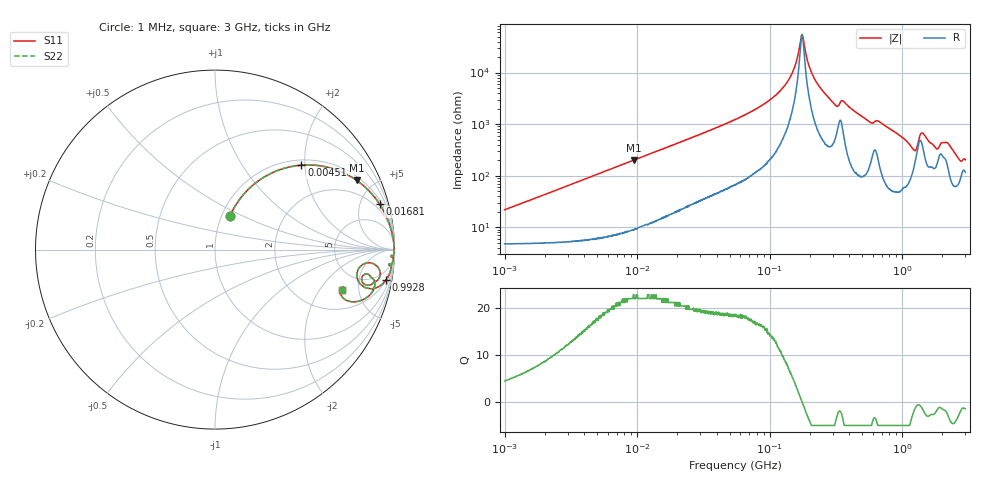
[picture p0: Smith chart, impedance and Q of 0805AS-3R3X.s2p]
!s-Parameter Generated by FASTRON Sdn. Bhd.
!FASTRON P/N : 0805AS-3R3X
!Keysight Technologies: E4991B_MY54100416_A.01.15
!Date: Mon Jun 15 12:58:39 2026
!Version  :Rev01  Mon Jun 15 12:58:39 2026
!Data & Calibration Information:
!Freq  S11  S21  S12  S22
!PortZ  Port1:50+j0  Port2:50+j0
!When reading reference impedance value at option line is always used.
! Remarks : This data is being provided solely for informational purposes.
# Hz S dB R 50
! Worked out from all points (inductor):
!   1601 points, 1 MHz to 3 GHz, reference 50 ohm
!   read as one part in series: L = 3.39 uH near 1.041 MHz
!   highest Q = 22.1 at 9.457 MHz (marker M1), where L = 3.38 uH
!   self-resonance near 175.8 MHz
!   S11 on the Smith chart (normalised r, x): 1 MHz: 1.10, +0.43; 4.51 MHz: 1.12, +1.92; 16.81 MHz: 1.33, +7.11; 992.8 MHz: 2, -11; 3 GHz: 3.32, -3.34
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1000000  -13.80 65.9  -0.58 -11.5  -0.58 -11.5  -13.80 65.9
3804036  -4.29 48.6  -2.47 -37.5  -2.47 -37.5  -4.29 48.6
4509552  -3.44 44.3  -3.09 -42.2  -3.09 -42.2  -3.44 44.3
9457300  -1.11 26.0  -7.17 -61.5  -7.17 -61.5  -1.11 26.0
1.447069e7  -0.55 17.8  -10.30 -69.6  -10.30 -69.6  -0.55 17.8
1.681455e7  -0.43 15.5  -11.50 -71.9  -11.50 -71.9  -0.43 15.5
5.504702e7  -0.07 4.6  -21.90 -82.3  -21.90 -82.3  -0.07 4.6
1.256933e8  -0.02 1.1  -34.10 -83.1  -34.10 -83.1  -0.02 1.1
1.512587e8  -0.02 0.5  -41.00 -77.6  -41.00 -77.6  -0.02 0.5
1.748812e8  -0.02 0.0  -54.70 -11.0  -54.70 -11.0  -0.02 0.0
2.083556e8  -0.02 -0.6  -39.70 78.8  -39.70 78.8  -0.02 -0.6
3.140564e8  -0.09 -2.4  -27.40 74.2  -27.40 74.2  -0.09 -2.4
3.594878e8  -0.08 -2.0  -29.00 74.1  -29.00 74.1  -0.08 -2.0
5.611759e8  -0.13 -5.0  -21.20 78.0  -21.20 78.0  -0.13 -5.0
7.925923e8  -0.13 -6.8  -18.60 79.4  -18.60 79.4  -0.13 -6.8
9.927591e8  -0.28 -9.9  -15.20 74.7  -15.20 74.7  -0.28 -9.9
1.231095e9  -1.50 -13.7  -11.40 47.4  -11.40 47.4  -1.50 -13.7
1.416254e9  -0.78 -6.2  -17.40 47.5  -17.40 47.5  -0.78 -6.2
1.782824e9  -1.18 -13.2  -12.10 53.0  -12.10 53.0  -1.18 -13.2
2.124078e9  -1.01 -10.2  -13.90 51.9  -13.90 51.9  -1.01 -10.2
2.660507e9  -1.79 -20.9  -8.49 50.5  -8.49 50.5  -1.79 -20.9
3e9  -2.56 -17.5  -8.73 37.7  -8.73 37.7  -2.56 -17.5
